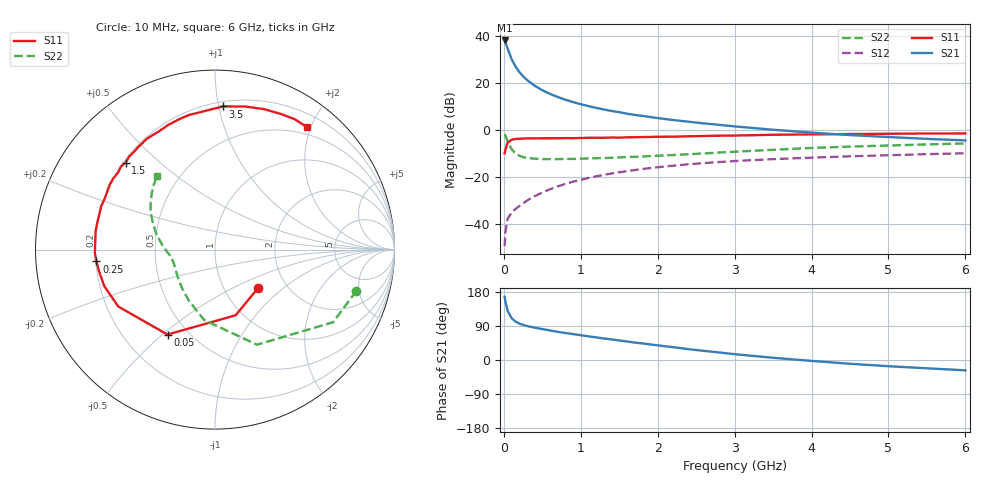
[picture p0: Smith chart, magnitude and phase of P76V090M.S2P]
! SIEMENS Small Signal Semiconductors
! BFP196
! Si NPN RF Bipolar Junction Transistor in SOT143
! VCE = 6 V  IC = 90 mA
! Common Emitter S-Parameters:  May  1996
# GHz  S  MA  R  50
!  f  S11  S21  S12  S22
! GHz  MAG  ANG  MAG  ANG  MAG  ANG  MAG  ANG
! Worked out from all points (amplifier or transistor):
!   36 points, 10 MHz to 6 GHz, reference 50 ohm
!   highest |S21| = 38.2 dB at 10 MHz (marker M1)
!   |S21| within 3 dB of that: start of sweep to 44.43 MHz
!   unconditionally stable (mu >= 1): 385.1 MHz to 4.695 GHz
!   at 250 MHz: K = 0.90, MSG = 27.0 dB, |S12| = -31.1 dB
!   at 1.4 GHz: K = 1.08, MAG = 11.5 dB, |S12| = -18.4 dB
!   at 6 GHz: K = 0.98, MSG = 2.7 dB, |S12| = -9.8 dB
!   S11 on the Smith chart (normalised r, x): 10 MHz: 1.45, -0.68; 50 MHz: 0.39, -0.52; 250 MHz: 0.20, -0.05; 1.5 GHz: 0.21, +0.39; 3.5 GHz: 0.23, +1.03; 6 GHz: 0.38, +1.94
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0.01  0.3215 -41.3  81.35 166.6  0.0034 81.0  0.8208 -16.3
0.02  0.3835 -72.5  74.67 154.0  0.0068 65.3  0.7724 -31.6
0.05  0.5423 -119.2  54.28 129.5  0.013 55.3  0.5791 -66.2
0.1  0.6251 -149.5  32.82 110.6  0.0177 50.3  0.3967 -98.8
0.15  0.6498 -161.8  22.89 101.7  0.0209 51.5  0.3204 -116.9
0.2  0.6568 -169.3  17.45 96.3  0.0242 55.2  0.2866 -128.7
0.25  0.6639 -174.3  13.99 92.6  0.0278 57.1  0.2677 -137.5
0.3  0.6697 -178.3  11.75 89.8  0.0317 60.0  0.2581 -143.3
0.4  0.6689 175.9  8.878 85.4  0.0394 62.9  0.2476 -151.8
0.5  0.6732 171.3  7.11 81.6  0.0471 64.3  0.2433 -157.4
0.6  0.673 166.8  5.926 78.0  0.0553 64.4  0.2421 -161.0
0.7  0.6743 162.6  5.092 74.3  0.0634 64.6  0.2428 -163.8
0.9  0.6769 155.4  3.965 68.4  0.0802 63.2  0.2451 -168.1
1.1  0.6892 148.3  3.259 62.4  0.0963 61.1  0.2506 -171.1
1.5  0.6948 135.8  2.419 51.5  0.1272 55.7  0.2636 -176.0
1.7  0.7077 129.3  2.118 46.0  0.1418 52.9  0.2715 -179.0
2.2  0.7282 115.9  1.645 33.8  0.1757 45.3  0.2963 174.7
2.8  0.7639 100.9  1.299 19.9  0.2105 36.2  0.3353 165.6
3.5  0.799 86.8  1.022 5.9  0.242 26.1  0.3831 155.5
4.5  0.8285 70.9  0.787 -9.9  0.2781 14.2  0.4477 143.2
5.5  0.8515 58.6  0.654 -21.9  0.3091 3.5  0.4984 133.1
6  0.8536 53.2  0.607 -27.3  0.3235 -2.3  0.5221 128.2
